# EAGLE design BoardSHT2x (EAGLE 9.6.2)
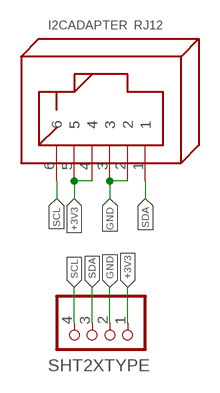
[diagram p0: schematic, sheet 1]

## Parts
I2CADAPTER  RJ12  [RJ12]
SHT2XTYPE  PINHD-1X4  [1X04]

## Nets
+3V3: I2CADAPTER.4 I2CADAPTER.5 SHT2XTYPE.1
GND: I2CADAPTER.2 I2CADAPTER.3 SHT2XTYPE.2
SCL: I2CADAPTER.6 SHT2XTYPE.4
SDA: I2CADAPTER.1 SHT2XTYPE.3

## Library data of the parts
I2CADAPTER = con-rj:RJ12: RJ12, RJ14 and RJ25 RJ12, RJ14 and RJ25 jacks side mounted http://www.tycoelectronics.com
SHT2XTYPE = pinhead:PINHD-1X4: PIN HEADER

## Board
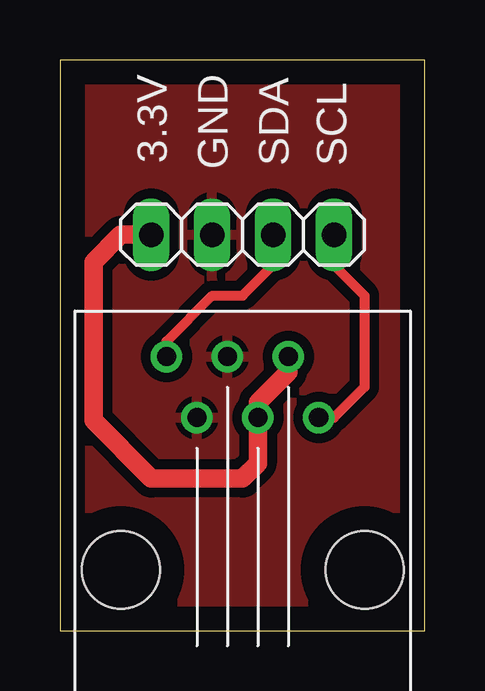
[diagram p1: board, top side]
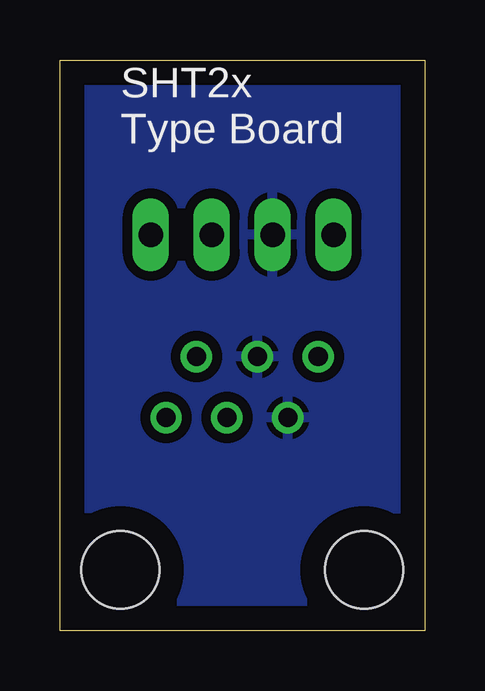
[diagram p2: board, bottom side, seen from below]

Size 15.22 x 23.8 mm. Coordinates in mm from the lower left corner, seen from the top.
Outline: 0,0 15.22,0 15.22,23.8 0,23.8 0,0
Copper layers (1*16): Top 0.035mm / dielectric 1.5mm / Bottom 0.035mm
Design rules "default": minimum track width 6mil, minimum drill 0.35mm, track to track 6mil, track to pad 6mil, pad to pad 6mil, via to via 6mil, smd to smd 6mil, copper to edge 40mil, drill to drill 6mil, minimum pad ring 10mil, minimum via ring 8mil, stop-mask expansion 4mil, vias tented up to drill 0mil, thermal gap 10mil

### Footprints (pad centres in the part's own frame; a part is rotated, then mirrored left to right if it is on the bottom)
RJ12 = drill 0.8: 1 -8.89,-3.175; 2 -6.35,-1.905; 3 -8.89,-0.635; 4 -6.35,0.635; 5 -8.89,1.905; 6 -6.35,3.175 | hole 3.25: 0,-5.08; 0,5.08
1X04 = drill 1.016 long: 1 -3.81,0; 2 -1.27,0; 3 1.27,0; 4 3.81,0

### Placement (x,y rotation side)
I2CADAPTER  7.62,2.54 270 top
SHT2XTYPE  7.62,16.51 0 top

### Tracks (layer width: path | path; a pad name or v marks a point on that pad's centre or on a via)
+3V3
  Top 0.762: I2CADAPTER.5 9.53,10.79 8.25,9.52 I2CADAPTER.4 8.25,6.98 7.62,6.35 3.81,6.35 1.4,8.76 1.4,15.37 2.54,16.51 SHT2XTYPE.1
GND
  pour Bottom (isolate 0.406): 0,24.13 15.24,24.13 15.24,0 0,0
  pour Top (isolate 0.406): 0,24.13 15.24,24.13 15.24,0 0,0
SCL
  Top 0.406: I2CADAPTER.6 11.43,8.89 12.7,10.16 12.7,13.97 11.43,15.24 SHT2XTYPE.4
SDA
  Top 0.406: I2CADAPTER.1 4.44,12.07 6.35,13.97 7.62,13.97 8.89,15.24 SHT2XTYPE.3

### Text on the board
tPlace: 3.3V | GND | SDA | SCL
bPlace: SHT2x / Type Board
